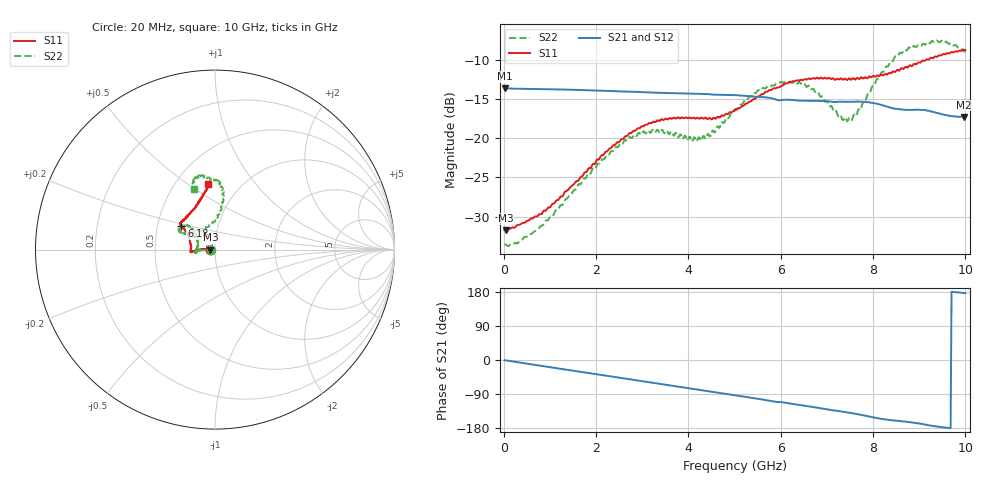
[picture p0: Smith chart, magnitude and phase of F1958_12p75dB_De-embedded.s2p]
! Integrated Device Technology
! Corporate Headquarters
! 6024 Silver Creek Valley Road
! San Jose, CA 95138  USA
! Phone:  1-408-284-8200
! Toll Free:  1-800-223-1366
! Webpage:  http://www.idt.com/
! Timing and RF Division
! 515 Groton Road, Suite 102
! Westford, MA 01886-6024
! Device:  F1958
! Description: 7-bit 0.25 dB Digital Step Attenuator
! Frequency:  0.001 -  6.000 GHz
! Package:  4x4 mm Thin QFN Plastic Package: 24 pin
! Ports:  2 RF, 12 DC
!  Pin  1  = D0
!  Pin  2  = VDD
!  Pin  3  = VMODE
!  Pin  4  = GND
!  Pin  5  = RF1  =  Port 1
!  Pin  6  = GND
!  Pin  7  = GND
!  Pin  8  = GND
!  Pin  9  = GND
!  Pin 10  = GND
!  Pin 11  = GND
!  Pin 12  = GND
!  Pin 13  = GND
!  Pin 14  = RF2  =  Port 2
!  Pin 15  = GND
!  Pin 16  = LE
!  Pin 17  = CLK
!  Pin 18  = DATA
!  Pin 19  = D6
!  Pin 20  = D5
!  Pin 21  = D4
!  Pin 22  = D3
!  Pin 23  = D2
!  Pin 24  = D1
! State:  51
! Atten State:  12.75 dB
! Voltage:  +3.30 Volts
! Current:  0.258 mA
! Data:  The device was measured on a F1958 evaluation board which has
!  individual transmission lines to the RF pins.  Data was collected
!  using a calibrated network analyzer.  The evaluation board was
!  de-embedded using Automatic Fixture Removal (AFR).
!  The reference plane is the edge of the package pin.
! Misc:
!  Action Tracker AT0419
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# GHz S dB R 50
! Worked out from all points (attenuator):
!   500 points, 20 MHz to 10 GHz, reference 50 ohm
!   highest |S21| = -13.59 dB at 20 MHz (marker M1); lowest = -17.2 dB at 9.96 GHz (marker M2)
!   lowest |S11| = -31.8 dB at 40 MHz (marker M3), VSWR 1.05, Z = 47.5 - j0.0834 ohm
!   |S11| at or under -10 dB: start of sweep to 9.132 GHz
!   |S22| runs from -33.8 to -7.5 dB; largest |S21 - S12| = 0.00063
!   S11 on the Smith chart (normalised r, x): 20 MHz: 0.95, -0.00; 6.18 GHz: 0.66, +0.18; 10 GHz: 0.71, +0.60
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0.02  -31.74 -178.1  -13.59 -0.5  -13.59 -0.5  -33.64 -177.8
0.04  -31.77 -178.1  -13.60 -0.9  -13.59 -0.9  -33.57 -176.8
0.32  -31.07 178.3  -13.64 -6.2  -13.64 -6.2  -33.32 179.5
0.72  -30.00 178.6  -13.68 -13.6  -13.67 -13.6  -31.69 -179.2
1.7  -24.88 178.9  -13.81 -31.8  -13.81 -31.8  -25.46 -179.4
2.6  -19.98 -178.2  -13.99 -48.5  -13.98 -48.5  -20.44 -175.8
3.36  -17.74 -174.1  -14.16 -62.5  -14.16 -62.6  -19.15 -169.6
4.24  -17.49 179.9  -14.29 -78.5  -14.30 -78.6  -19.90 167.7
4.5  -17.57 174.0  -14.38 -83.6  -14.39 -83.6  -19.32 152.3
5.02  -16.41 159.3  -14.46 -93.1  -14.47 -93.1  -16.22 138.6
5.54  -14.59 149.1  -14.69 -103.0  -14.70 -103.0  -13.83 139.6
6.18  -12.82 145.2  -15.06 -114.5  -15.07 -114.5  -12.79 148.7
6.68  -12.31 142.4  -15.20 -123.6  -15.21 -123.5  -13.69 152.2
7.3  -12.31 136.1  -15.30 -135.5  -15.31 -135.3  -17.03 130.1
7.5  -12.37 133.3  -15.32 -139.4  -15.32 -139.3  -17.33 111.7
7.68  -12.34 130.3  -15.28 -143.3  -15.28 -143.3  -16.31 95.2
8.34  -11.63 114.6  -16.00 -158.1  -16.00 -158.2  -10.63 80.7
8.68  -10.99 107.8  -16.34 -162.4  -16.34 -162.3  -8.64 85.4
9.28  -9.73 100.0  -16.58 -173.9  -16.59 -173.9  -7.50 99.8
9.58  -9.20 96.8  -17.02 -178.5  -17.04 -178.6  -7.61 105.0
9.96  -8.63 96.2  -17.24 176.9  -17.25 176.9  -8.81 108.9
10  -8.69 96.1  -17.21 176.1  -17.24 176.2  -8.95 109.1
